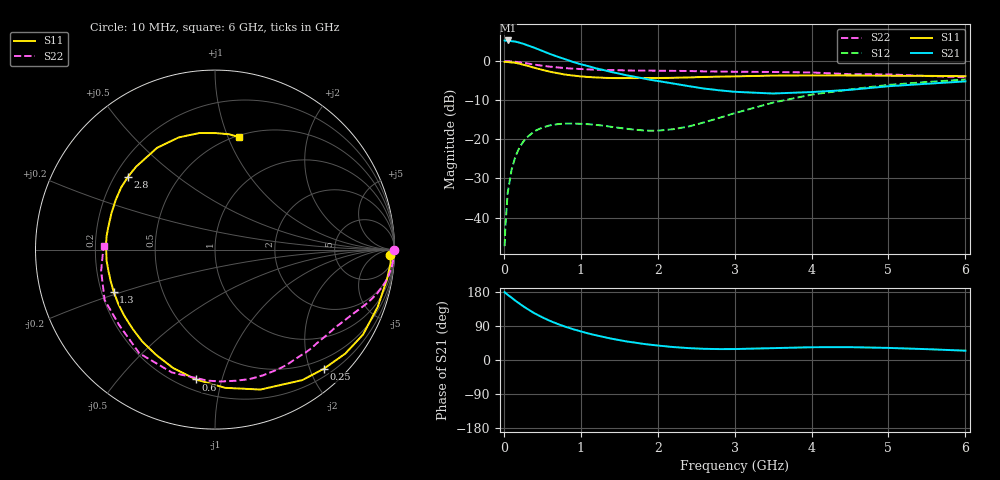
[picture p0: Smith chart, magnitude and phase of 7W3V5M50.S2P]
! Infineon Technologies  Discrete & RF Semiconductors
! BFS17W
! Si NPN RF Bipolar Junction Transistor in SOT323
! VCE = 3.5 V  IC = 0.5 mA
! Common Emitter S-Parameters:  August  1999
# GHz  S  MA  R  50
!  f  S11  S21  S12  S22
! GHz  MAG  ANG  MAG  ANG  MAG  ANG  MAG  ANG
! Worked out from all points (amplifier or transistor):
!   36 points, 10 MHz to 6 GHz, reference 50 ohm
!   highest |S21| = 5.3 dB at 50 MHz (marker M1)
!   |S21| within 3 dB of that: start of sweep to 542.3 MHz
!   unconditionally stable (mu >= 1): 1.203 GHz to end of sweep
!   at 250 MHz: K = 0.22, MSG = 12.6 dB, |S12| = -20.7 dB
!   at 1.4 GHz: K = 1.16, MAG = 4.6 dB, |S12| = -16.8 dB
!   at 6 GHz: K = 1.10, MAG = -2.1 dB, |S12| = -4.7 dB
!   S11 on the Smith chart (normalised r, x): 10 MHz: 28, -41; 250 MHz: 0.32, -2.23; 600 MHz: 0.27, -0.83; 1.3 GHz: 0.25, -0.19; 2.8 GHz: 0.25, +0.34; 6 GHz: 0.52, +1.10
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0.01  0.9774 -1.9  1.834 179.2  0.0043 89.8  0.9999 -0.1
0.02  0.9819 -4.3  1.826 177.0  0.0076 87.2  0.9975 -1.1
0.05  0.9722 -9.9  1.836 172.0  0.0206 84.4  0.9958 -2.9
0.1  0.9612 -19.4  1.798 164.6  0.0406 78.4  0.9896 -5.7
0.15  0.9509 -29.9  1.775 156.5  0.0602 71.7  0.9786 -8.4
0.25  0.8992 -47.6  1.669 142.2  0.0926 61.6  0.9496 -13.2
0.3  0.8749 -56.2  1.602 135.5  0.1058 57.1  0.9343 -15.3
0.4  0.8198 -72.0  1.477 123.1  0.1272 48.6  0.9019 -19.1
0.5  0.7722 -85.8  1.351 112.7  0.1411 42.0  0.8719 -22.2
0.6  0.7314 -98.4  1.233 103.2  0.1509 36.7  0.8486 -24.9
0.8  0.6719 -119.3  1.056 87.8  0.1591 28.8  0.8131 -30.2
1.1  0.6256 -143.9  0.86 69.9  0.156 22.7  0.783 -37.7
1.3  0.6115 -157.4  0.767 60.6  0.1494 21.4  0.7703 -43.0
1.6  0.6073 -174.0  0.657 48.8  0.1363 24.3  0.7592 -51.1
2.2  0.6114 160.7  0.517 34.2  0.1345 45.0  0.75 -68.8
2.8  0.6322 139.9  0.423 28.8  0.1877 61.8  0.7356 -87.6
3.5  0.6525 119.6  0.385 31.3  0.2948 63.1  0.7255 -109.3
4  0.6569 107.9  0.402 33.7  0.3722 57.4  0.7153 -126.1
4.5  0.6553 97.6  0.429 33.9  0.4341 50.4  0.6796 -141.7
5  0.6492 89.7  0.477 31.9  0.4966 43.4  0.6762 -155.4
5.5  0.6474 83.0  0.513 28.6  0.5406 36.6  0.6455 -169.4
6  0.6406 77.8  0.55 24.6  0.58 30.3  0.6212 178.4
